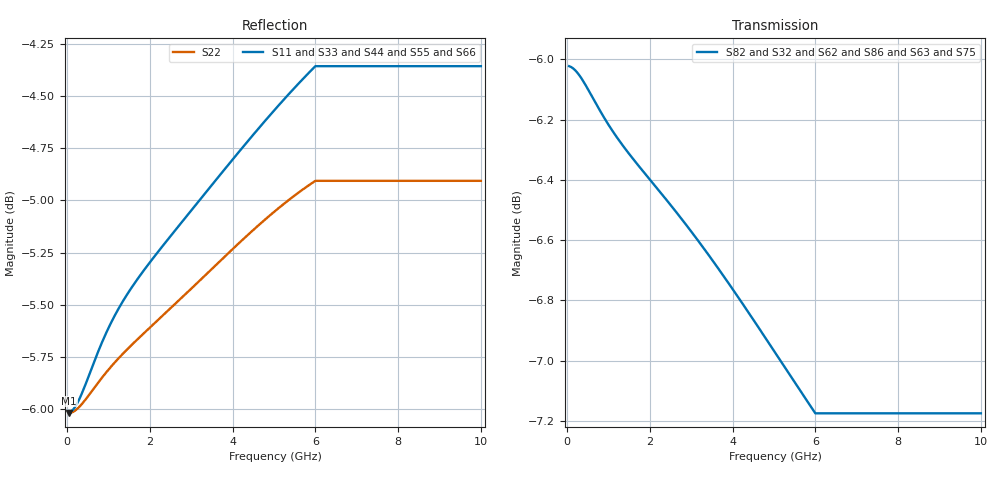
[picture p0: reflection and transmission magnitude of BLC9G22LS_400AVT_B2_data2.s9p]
! Created Tue Aug  4 10:32:27 2015
# ghz S ma R 50
! 9 Port Network Data from SP1.SP block
! freq  magS11  angS11  magS12  angS12  magS13  angS13  magS14  angS14
!  magS15  angS15  magS16  angS16  magS17  angS17  magS18  angS18
!  magS19  angS19
!  magS21  angS21  magS22  angS22  magS23  angS23
!  magS24  angS24  magS25  angS25  magS26  angS26  magS27  angS27
!  magS28  angS28  magS29  angS29
!  magS31  angS31  magS32  angS32
!  magS33  angS33  magS34  angS34  magS35  angS35  magS36  angS36
!  magS37  angS37  magS38  angS38  magS39  angS39
!  magS41  angS41
!  magS42  angS42  magS43  angS43  magS44  angS44  magS45  angS45
!  magS46  angS46  magS47  angS47  magS48  angS48  magS49  angS49
!  magS51  angS51  magS52  angS52  magS53  angS53  magS54  angS54
!  magS55  angS55  magS56  angS56  magS57  angS57  magS58  angS58
!  magS59  angS59
!  magS61  angS61  magS62  angS62  magS63  angS63
!  magS64  angS64  magS65  angS65  magS66  angS66  magS67  angS67
!  magS68  angS68  magS69  angS69
!  magS71  angS71  magS72  angS72
!  magS73  angS73  magS74  angS74  magS75  angS75  magS76  angS76
!  magS77  angS77  magS78  angS78  magS79  angS79
!  magS81  angS81
!  magS82  angS82  magS83  angS83  magS84  angS84  magS85  angS85
!  magS86  angS86  magS87  angS87  magS88  angS88  magS89  angS89
!  magS91  angS91  magS92  angS92  magS93  angS93  magS94  angS94
!  magS95  angS95  magS96  angS96  magS97  angS97  magS98  angS98
!  magS99  angS99
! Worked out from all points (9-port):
!   200 points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, 50 MHz to 10 GHz, reference 50 ohm
!   strongest paths, dB at 50 MHz, 2.55 GHz, 5.05 GHz, 7.55 GHz, 10 GHz:
!     S82: -6.0, -6.5, -7.0, -7.2, -7.2
!     S32: -6.0, -6.5, -7.0, -7.2, -7.2
!     S62: -6.0, -6.5, -7.1, -7.3, -7.3
!     S86: -6.0, -6.5, -7.1, -7.4, -7.4
!     S63: -6.0, -6.5, -7.1, -7.4, -7.4
!     S75: -6.0, -6.8, -7.3, -7.5, -7.5
!   lowest |S11| = -6.0 dB at 50 MHz (marker M1), VSWR 3.00, Z = 16.7 - j0.128 ohm
!   |S11| at or under -10 dB: nowhere
